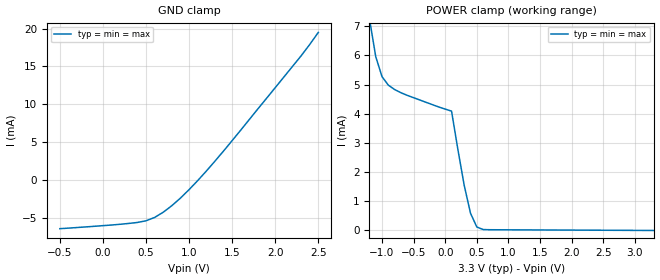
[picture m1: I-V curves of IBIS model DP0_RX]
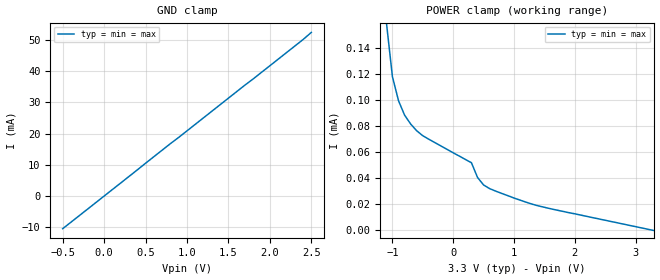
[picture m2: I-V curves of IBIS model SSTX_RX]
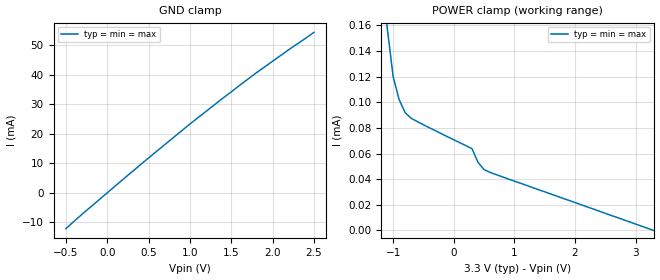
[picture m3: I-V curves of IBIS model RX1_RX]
|   Texas Instruments Incorporated
|   High Speed Interface Products
|   IBIS Model for TUSB1146
|   40PIN RNQ Package
[IBIS Ver]   6.0
[Comment char]   |_char
[File name]   tusb1146.ibs
[File Rev]   1.0
[Date]   Mon Nov 18 19:21:15 2019
[Source]   File originated at Texas Instruments Incorporated.
   Data Transmission Products Group. All data based on
   Simulation Measurements.
[Notes]
[Disclaimer]
(C) Copyright Texas Instruments Incorporated 2019
   All rights reserved
  Texas Instruments Incorporated hereby grants the user of this IBIS
model a non-exclusive, nontransferable license to use this IBIS model
under the following terms.  Before using this IBIS model, the user
should read this license.  If the user does not accept these terms,
the IBIS model should be returned to Texas Instruments within 30 days.
  The user is granted this license only to use the IBIS model and
is not granted rights to sell, load, rent, lease or license the IBIS
model in whole or in part, or in modified form to anyone other than
user.  User may modify the IBIS model to suit its specific applications
but rights to derivative works and such modifications shall belong to
Texas Instruments.
  This IBIS model is provided on an "AS IS" basis and Texas Instruments
makes absolutely no warranty with respect to the information contained
herein.  TEXAS INSTRUMENTS DISCLAIMS AND CUSTOMER WAIVES ALL WARRANTIES,
EXPRESS OR IMPLIED, INCLUDING WARRANTIES OF MERCHANTABILITY OR FITNESS
FOR A PARTICULAR PURPOSE. The entire risk as to quality and performance
is with the Customer. ACCORDINGLY, IN NO EVENT SHALL THE COMPANY BE LIABLE
FOR ANY DAMAGES, WHETHER IN CONTRACT OR TORT,INCLUDING ANY LOST PROFITS
OR OTHER INCIDENTAL, CONSEQUENTIAL, EXEMPLARY, OR PUNITIVE DAMAGES ARISING
OUT OF THE USE OR APPLICATION OF THE IBIS model provided in this package.
Further, Texas Instruments reserves the right to discontinue or make changes
without notice to any product herein to improve reliability, function, or
design. Texas Instruments does not convey any license under patent rights
or any other intellectual property rights, including those of third parties.
Contact Texas Instruments at ATTN:DATA TRANSMISSIONS
[Copyright]   Copyright 2019, Texas Instruments, All Rights Reserved
[Component]   TUSB1146
[Manufacturer]  Texas Instruments Incorporated
[Package]
R_pkg 0.083 0.065 0.101
L_pkg 1.4245e-09 1.118e-9 1.731e-9
C_pkg 2.195e-13 0.195e-12 0.244e-12
[Pin]   signal_name   model_name   R_pin	L_pin		C_pin
1 VCC POWER 0.091 1.624e-9 0.219e-12
4 SSRXN SSRX_TX 0.076 1.367e-9 0.219e-12
5 SSRXP SSRX_TX 0.074 1.391e-9 0.216e-12
6 VCC POWER 0.076 1.431e-9 0.215e-12
7 SSTXN SSTX_RX 0.080 1.521e-9 0.229e-12
8 SSTXP SSTX_RX 0.089 1.661e-9 0.216e-12
9 DP0P DP0_RX 0.091 1.626e-9 0.217e-12
10 DP0N DP0_RX 0.082 1.419e-9 0.233e-12
20 VCC POWER 0.097 1.713e-9 0.240e-12
28 VCC POWER 0.089 1.667e-9 0.216e-12
30 RX1N RX1_RX 0.093 1.586e-9 0.244e-12
31 RX1P RX1_RX 0.085 1.473e-9 0.226e-12
33 TX1N TX1_TX 0.073 1.296e-9 0.209e-12
34 TX1P TX1_TX 0.068 1.207e-9 0.202e-12
39 RX2N RX2_TX 0.076 1.390e-9 0.213e-12
40 RX2P RX2_TX 0.084 1.573e-9 0.207e-12
|9	 DP0P   DP0_RX   0.091	0.704e-9	0.137e-12
|10	 DP0N   DP0_RX   0.091	0.704e-9	0.137e-12
|12	 DP1P   DP1_RX   0.091	0.704e-9	0.137e-12
|13	 DP1N   DP1_RX   0.091	0.704e-9	0.137e-12
|15	 DP2P   DP2_RX   0.091	0.704e-9	0.137e-12
|16	 DP2N   DP2_RX   0.091	0.704e-9	0.137e-12
|18	 DP3P   DP3_RX   0.091	0.704e-9	0.137e-12
|19	 DP3N   DP3_RX   0.091	0.704e-9	0.137e-12
|31 	 RX1P   RX1   0.091	0.704e-9	0.137e-12
|30   RX1N   RX1   0.091 	0.704e-9 	0.137e-12
|40 	 RX2P   RX2   0.091	0.704e-9	0.137e-12
|39   RX2N   RX2   0.091 	0.704e-9 	0.137e-12
|34 	 TX1P   TX1_TX   0.091	0.704e-9	0.137e-12
|33   TX1N   TX1_TX   0.091 	0.704e-9 	0.137e-12
|37 	 TX2P   TX2_TX   0.091	0.704e-9	0.137e-12
|36   TX2N   TX2_TX   0.091 	0.704e-9 	0.137e-12
|8   SSTXP   SSTX_RX   0.091 	0.704e-9 	0.137e-12
|7   SSTXN   SSTX_RX   0.091 	0.704e-9 	0.137e-12
|5   SSRXP   SSRX_TX   0.091 	0.704e-9 	0.137e-12
|4   SSRXN   SSRX_TX   0.091 	0.704e-9 	0.137e-12
|1   VCC   POWER   0.091 	0.704e-9 	0.137e-12
|6   VCC   POWER   0.091 	0.704e-9 	0.137e-12
|20   VCC   POWER   0.091 	0.704e-9 	0.137e-12
|28   VCC   POWER   0.091 	0.704e-9 	0.137e-12
THPAD	 GND   GND   0.001	0.100e-9	1.000e-12
[Diff_pin]   inv_pin   vdiff   tdelay_typ   tdelay_min   tdelay_max
5 4 0 0 0 0
8 7 0.0 0 0 0
9 10 0.0 0 0 0
31 30 0.0 0 0 0
34 33 0.0 0 0 0
40 39 0.0 0 0 0
| Models and submodels in the file (6): DP0_RX (Input), SSTX_RX (Input), RX1_RX (Input), RX2_TX (Output), TX1_TX (Output), SSRX_TX (Output)
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|9   10   NA   NA   NA   NA
|12   13   NA   NA   NA   NA
|15   16   NA   NA   NA   NA
|18   19   NA   NA   NA   NA
|31   30   NA   NA   NA   NA
|40   39   NA   NA   NA   NA
|34   33   NA   NA   NA   NA
|37   36   NA   NA   NA   NA
|8   7   NA   NA   NA   NA
|5   4   NA   NA   NA   NA
|[Repeater Pin] tx_non_inv_pin
|15 34
|9 31
|[Model Selector] RX1
|RX1_TX   TX model for the bi-directional RX1 pins
|RX1_RX		 RX model for the bi-directional RX1 pins
|[Model Selector] RX2
|RX2_TX   TX model for the bi-directional RX2 pins
|RX2_RX		 RX model for the bi-directional RX2 pins
[Model]   DP0_RX
Model_type   Input
Vinh=1.9
Vinl=1.7
| typ min max
C_comp 0.167p 0.167p 0.167p
[Algorithmic Model]
Executable Windows_cl19.00.24215.1_64  DP0_RX_x64.dll DP0_RX.ami
Executable Linux_gcc5.4.0_64 DP0_RX_x64.so DP0_RX.ami
[End Algorithmic Model]
[Temperature Range] 27.0 27.0 27.0
[Voltage range] 3.3 3.3 3.3
[GND_clamp]
|   Voltage   I(typ)   I(min)   I(max)
-500mV    -6.44mA    -6.44mA    -6.44mA
400mV     -5.62mA    -5.62mA    -5.62mA
500mV     -5.4mA     -5.4mA     -5.4mA
600mV     -4.96mA    -4.96mA    -4.96mA
700mV     -4.27mA    -4.27mA    -4.27mA
800mV     -3.4mA     -3.4mA     -3.4mA
1V        -1.28mA    -1.28mA    -1.28mA
1.3V      2.48mA     2.48mA     2.48mA
2.3V      16.4mA     16.4mA     16.4mA
2.5V      19.5mA     19.5mA     19.5mA
| Note that the[POWER_clamp]voltage table is referenced to Vcc
| and is calculated using Vtable=Vcc - Vmeasured.
|   Voltage   I(typ)   I(min)   I(max)
[Power_clamp]
-1.7V     23.7mA     23.7mA     23.7mA
-1.2V     7.27mA     7.27mA     7.27mA
-1.1V     5.96mA     5.96mA     5.96mA
-1V       5.27mA     5.27mA     5.27mA
-900mV    4.98mA     4.98mA     4.98mA
-600mV    4.63mA     4.63mA     4.63mA
100mV     4.09mA     4.09mA     4.09mA
300mV     1.55mA     1.55mA     1.55mA
400mV     591uA      591uA      591uA
500mV     118uA      118uA      118uA
700mV     25.7uA     25.7uA     25.7uA
3.3V      -111nA     -111nA     -111nA
[Model]   SSTX_RX
Model_type   Input
Vinh=0.1
Vinl=-0.1
| typ min max
C_comp 0.269p 0.269p 0.269p
[Algorithmic Model]
Executable Windows_cl19.00.24215.1_64  SSTX_RX_x64.dll SSTX_RX.ami
Executable Linux_gcc5.4.0_64 SSTX_RX_x64.so SSTX_RX.ami
[End Algorithmic Model]
[Temperature Range] 27.0 27.0 27.0
[Voltage range] 3.3 3.3 3.3
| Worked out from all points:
|   GND clamp passes 1 mA (typ) near -0.05 V on its own axis
|   POWER clamp passes 1 mA (typ) near -1.34 V on its own axis
[GND_clamp]
|   Voltage   I(typ)   I(min)   I(max)
-500mV    -10.5mA    -10.5mA    -10.5mA
2V        41.8mA     41.8mA     41.8mA
2.4V      50.2mA     50.2mA     50.2mA
2.5V      52.5mA     52.5mA     52.5mA
| Note that the[POWER_clamp]voltage table is referenced to Vcc
| and is calculated using Vtable=Vcc - Vmeasured.
|   Voltage   I(typ)   I(min)   I(max)
[Power_clamp]
-1.7V     31.1mA     31.1mA     31.1mA
-1.1V     160uA      160uA      160uA
-1V       118uA      118uA      118uA
-900mV    99.6uA     99.6uA     99.6uA
-800mV    88.5uA     88.5uA     88.5uA
-700mV    81.7uA     81.7uA     81.7uA
-500mV    72.7uA     72.7uA     72.7uA
300mV     52uA       52uA       52uA
400mV     40.7uA     40.7uA     40.7uA
500mV     34.9uA     34.9uA     34.9uA
1.4V      18.9uA     18.9uA     18.9uA
3.3V      -126pA     -126pA     -126pA
[Model]   RX1_RX
Model_type   Input
Vinh=0.1
Vinl=-0.1
| typ min max
C_comp 0.404p 0.404p 0.404p
[Algorithmic Model]
Executable Windows_cl19.00.24215.1_64  RX1_RX_x64.dll RX1_RX.ami
Executable Linux_gcc5.4.0_64 RX1_RX_x64.so RX1_RX.ami
[End Algorithmic Model]
[Temperature Range] 27.0 27.0 27.0
[Voltage range] 3.3 3.3 3.3
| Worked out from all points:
|   GND clamp passes 1 mA (typ) near -0.04 V on its own axis
|   POWER clamp passes 1 mA (typ) near -1.34 V on its own axis
[GND_clamp]
|   Voltage   I(typ)   I(min)   I(max)
-500mV    -12.2mA    -12.2mA    -12.2mA
200mV     4.74mA     4.74mA     4.74mA
1V        23.3mA     23.3mA     23.3mA
1.8V      40.6mA     40.6mA     40.6mA
2.5V      54.4mA     54.4mA     54.4mA
| Note that the[POWER_clamp]voltage table is referenced to Vcc
| and is calculated using Vtable=Vcc - Vmeasured.
|   Voltage   I(typ)   I(min)   I(max)
[Power_clamp]
-1.7V     31.1mA     31.1mA     31.1mA
-1.1V     159uA      159uA      159uA
-1V       120uA      120uA      120uA
-900mV    102uA      102uA      102uA
-800mV    91.8uA     91.8uA     91.8uA
-700mV    87.5uA     87.5uA     87.5uA
-600mV    84.9uA     84.9uA     84.9uA
300mV     63.9uA     63.9uA     63.9uA
400mV     53.2uA     53.2uA     53.2uA
500mV     47.5uA     47.5uA     47.5uA
1V        38.5uA     38.5uA     38.5uA
3.3V      -18.2pA    -18.2pA    -18.2pA
